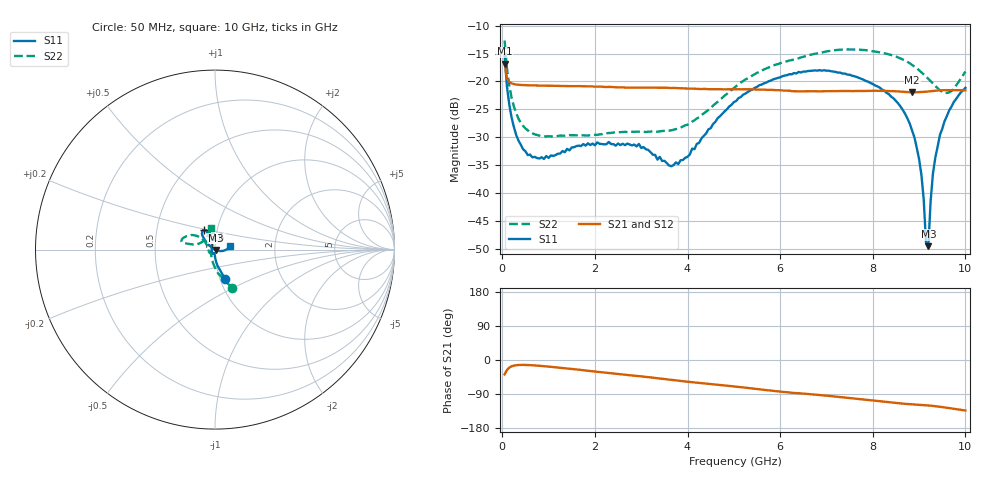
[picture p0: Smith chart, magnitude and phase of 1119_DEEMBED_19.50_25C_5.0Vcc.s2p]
!Hittite Microwave Corp.
!Digital Attenuator/PhaseShifter Rev 1.4.0
!Filename: C:\DATA\DATA\1119_DEEMBED_19.50_25C_5.0Vcc.s2p
!VNA ID: Agilent Technologies,N5224A,MY51441122,A.10.45.03
!Device type:
!2 Port Calibration.
!Temp(C): 25
!Lot Number:
!Serial Number:
!Operator:
!Misc:
!Attenuator:  19.500
# GHZ S DB R 50.0
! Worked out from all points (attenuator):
!   200 points, 50 MHz to 10 GHz, reference 50 ohm
!   highest |S21| = -16.83 dB at 50 MHz (marker M1); lowest = -21.9 dB at 8.85 GHz (marker M2)
!   lowest |S11| = -49.5 dB at 9.2 GHz (marker M3), VSWR 1.01, Z = 50.3 - j0.143 ohm
!   |S11| at or under -10 dB: start of sweep to end of sweep
!   |S22| runs from -29.9 to -12.7 dB; largest |S21 - S12| = 0.0003
!   S11 on the Smith chart (normalised r, x): 50 MHz: 1.06, -0.35; 6.6 GHz: 0.87, +0.19; 10 GHz: 1.18, +0.05
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0.05  -15.37 -71.2  -16.83 -38.0  -16.83 -38.1  -12.66 -66.0
0.1  -20.86 -81.2  -19.36 -26.4  -19.36 -26.3  -17.60 -83.1
0.2  -26.44 -88.3  -20.33 -16.7  -20.33 -16.7  -22.88 -99.8
0.55  -33.19 -99.2  -20.69 -13.2  -20.68 -13.3  -28.76 -125.3
1.75  -31.22 -122.1  -20.86 -26.9  -20.86 -27.0  -29.65 -138.9
2.95  -31.19 -131.3  -21.09 -42.5  -21.10 -42.6  -29.00 -158.0
3.4  -33.51 -156.1  -21.12 -48.8  -21.12 -48.8  -28.94 -171.2
3.8  -34.80 161.4  -21.20 -54.6  -21.20 -54.6  -28.43 173.0
5.05  -23.50 110.4  -21.40 -70.3  -21.42 -70.4  -20.85 140.0
6.6  -18.14 119.1  -21.76 -89.7  -21.78 -89.7  -15.35 153.7
6.7  -18.08 120.2  -21.75 -90.8  -21.76 -90.8  -15.14 154.8
8.35  -22.28 136.7  -21.72 -111.3  -21.73 -111.3  -15.15 167.9
8.85  -28.80 142.6  -21.95 -116.9  -21.95 -116.9  -17.04 167.5
9.05  -36.69 148.7  -21.89 -118.5  -21.90 -118.5  -18.35 166.5
9.1  -41.13 148.8  -21.87 -118.9  -21.89 -118.9  -18.74 165.8
9.15  -48.90 156.9  -21.84 -119.4  -21.85 -119.4  -19.13 164.9
9.2  -49.50 -25.1  -21.79 -119.9  -21.81 -120.0  -19.55 163.6
9.25  -41.39 -23.2  -21.76 -120.5  -21.78 -120.5  -19.96 161.8
9.3  -36.44 -21.4  -21.71 -121.2  -21.73 -121.2  -20.36 159.6
9.45  -29.58 -15.0  -21.59 -123.4  -21.60 -123.4  -21.60 149.2
9.7  -24.51 -2.4  -21.55 -127.8  -21.56 -127.8  -21.70 121.3
10  -21.15 14.2  -21.58 -133.2  -21.59 -133.2  -18.23 99.8
